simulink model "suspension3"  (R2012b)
settings: Solver=ode45  StartTime=0.0  StopTime=10.0  RelTol=1e-3
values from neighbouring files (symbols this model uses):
  a11y = a{1,:}    [suspension_2.m]    (also in suspension_3.m)
  a11z = a{1,:}    [suspension_2.m]    (also in suspension_3.m)
  b11y = b{1,:}    [suspension_2.m]    (also in suspension_3.m)
  b11z = b{1,:}    [suspension_2.m]    (also in suspension_3.m)
  b12y = b{2,:}    [suspension_2.m]    (also in suspension_3.m)
  b12z = b{2,:}    [suspension_2.m]    (also in suspension_3.m)
  b13y = b{3,:}    [suspension_2.m]    (also in suspension_3.m)
  b13z = b{3,:}    [suspension_2.m]    (also in suspension_3.m)
  b14y = b{4,:}    [suspension_2.m]    (also in suspension_3.m)
  b14z = b{4,:}    [suspension_2.m]    (also in suspension_3.m)
  delay = (L/v)    (= 0.1)    [suspension_2.m]    (also in suspension_3.m)
  dt = 0.001    [coulomb_1.m]    (also in coulomb_10.m; coulomb_11.m; coulomb_2.m; coulomb_3.m)
  Fs = 1/dt    (= 500)    [unwucht_rueckw_1.m]
  varianz = 1e-6    (= 1e-06)    [diff_filter_1.m]    (also in diff_filter_2.m = 1e-08; rad_aufhaeng_4.m = 2e-06; suspension_2.m = 2e-06; suspension_3.m = 2e-06)
undefined symbols (not defined in the file or in its folder): dBW, get, Hertz, sided, Two
libraries: dspsnks4 x1

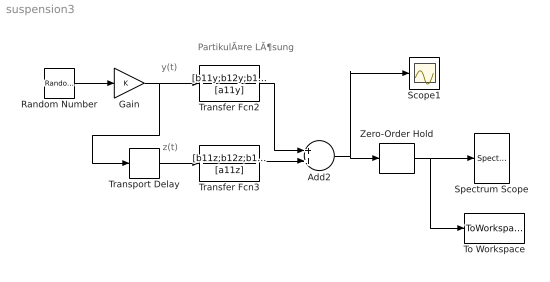
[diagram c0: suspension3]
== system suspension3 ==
  note: z(t)
  note: y(t)
  note: PartikulÃ¤re LÃ¶sung
  Add2 : Sum
  Gain : Gain
  Random Number : RandomNumber  Variance=varianz  Seed=1395  SampleTime=dt
  Scope1 : Scope
  Spectrum Scope : dspsnks4/Spectrum Scope  ScopeProperties=on  Domain=Frequency  HorizSpan=1  UseBuffer=on  BufferSize=128  Overlap=0  TreatMby1Signals=M channels  inpFftLenInherit=off  FFTlength=128  numAvg=100  DisplayProperties=off  AxisGrid=on  Memory=off  FrameNumber=on  AxisLegend=off  AxisZoom=off  OpenScopeAtSimStart=on  OpenScopeImmediately=off  FigPos=get(0,'defaultfigureposition')  AxisProperties=off  XUnits=Hertz  XRange=Two-sided ((-Fs/2...Fs/2])  XDisplay=0  InheritXIncr=on  XIncr=1.0  XLabel=Samples  XLimit=User-defined  YUnits=dBW/Hertz  XMax=50  XMin=-50  YLabel=Magnitude-squared, dB  LineProperties=off  LineStyles=-|--|:|-.  LineMarkers=*|.|x|o  wintypeSpecScope=Hann  RsSpecScope=50  betaSpecScope=5  winsampSpecScope=Periodic  XAxisParamsVer=6.9  isFrameUpgraded=on
  To Workspace : ToWorkspace  VariableName=y  SampleTime=-1  SaveFormat=Structure With Time
  Transfer Fcn2 : TransferFcn  Numerator=[b11y;b12y;b13y;b14y]  Denominator=[a11y]
  Transfer Fcn3 : TransferFcn  Numerator=[b11z;b12z;b13z;b14z]  Denominator=[a11z]
  Transport Delay : TransportDelay  DelayTime=delay
  Zero-Order Hold : ZeroOrderHold  SampleTime=dt
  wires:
  Transfer Fcn2/1 -> Add2/1
  Transfer Fcn3/1 -> Add2/2
  Transport Delay/1 -> Transfer Fcn3/1
  Random Number/1 -> Gain/1
  Gain/1 -> Transport Delay/1, Transfer Fcn2/1
  Add2/1 -> Scope1/1, Zero-Order Hold/1
  Zero-Order Hold/1 -> To Workspace/1, Spectrum Scope/1
